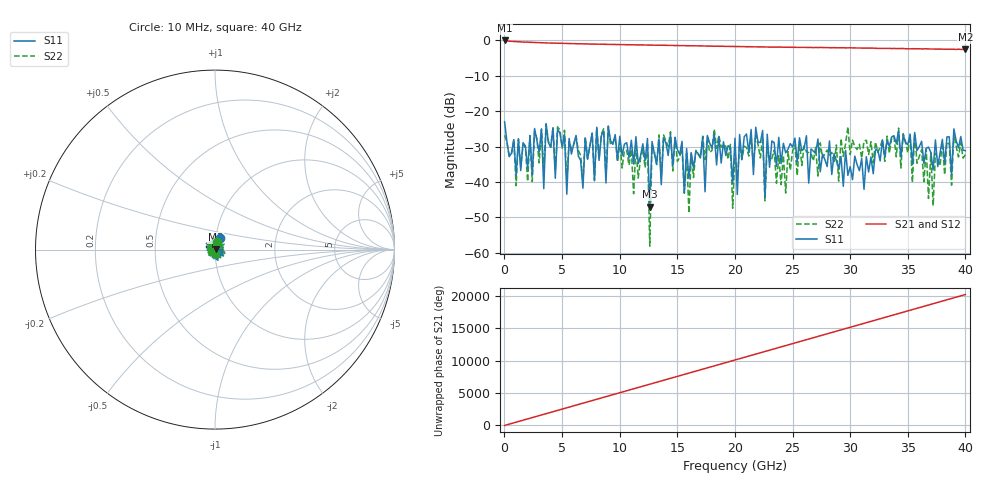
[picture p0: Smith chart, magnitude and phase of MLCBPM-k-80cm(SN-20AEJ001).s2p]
!Keysight Technologies,N5225A,MY51451228,A.10.40.14
!Date: Friday, November 20, 2020 11:31:11
!Correction: S11(Full 2 Port(1,2))
!S21(Full 2 Port(1,2))
!S12(Full 2 Port(1,2))
!S22(Full 2 Port(1,2))
!S2P File: Measurements: S11, S21, S12, S22:
# Hz S  dB  R 50
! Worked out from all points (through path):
!   201 points, 10 MHz to 40 GHz, reference 50 ohm
!   highest |S21| = -0.04 dB at 10 MHz (marker M1); lowest = -2.6 dB at 40 GHz (marker M2)
!   lowest |S11| = -46.9 dB at 12.61 GHz (marker M3), VSWR 1.01, Z = 50.4 + j0.142 ohm
!   |S11| at or under -10 dB: start of sweep to end of sweep
!   |S22| runs from -58.1 to -23.7 dB; largest |S21 - S12| = 0.014
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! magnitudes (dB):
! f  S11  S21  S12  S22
! 10 MHz  -23.0  0.0  -0.1  -26.8
! 6.808 GHz  -41.8  -1.0  -1.0  -40.2
! 12.41 GHz  -27.7  -1.3  -1.3  -29.2
! 12.61 GHz  -46.9  -1.3  -1.4  -58.1
! 12.81 GHz  -28.6  -1.4  -1.4  -29.6
! 13.41 GHz  -27.9  -1.4  -1.4  -26.7
! 15.81 GHz  -30.6  -1.5  -1.5  -31.9
! 16.01 GHz  -39.0  -1.5  -1.5  -48.8
! 17.21 GHz  -27.2  -1.6  -1.6  -27.1
! 17.41 GHz  -42.8  -1.6  -1.6  -33.7
! 17.61 GHz  -26.9  -1.6  -1.6  -27.4
! 19.61 GHz  -30.2  -1.7  -1.7  -29.4
! 19.81 GHz  -40.4  -1.7  -1.7  -47.4
! 20 GHz  -27.6  -1.8  -1.8  -31.3
! 20.2 GHz  -43.5  -1.8  -1.8  -39.7
! 20.4 GHz  -26.6  -1.8  -1.8  -29.6
! 22.4 GHz  -25.5  -1.9  -1.9  -27.2
! 22.6 GHz  -44.5  -1.9  -1.9  -45.3
! 22.8 GHz  -26.5  -1.9  -1.9  -29.4
! 26.8 GHz  -31.3  -2.1  -2.0  -34.1
! 33.4 GHz  -29.9  -2.3  -2.3  -31.9
! 40 GHz  -31.2  -2.6  -2.6  -32.3
